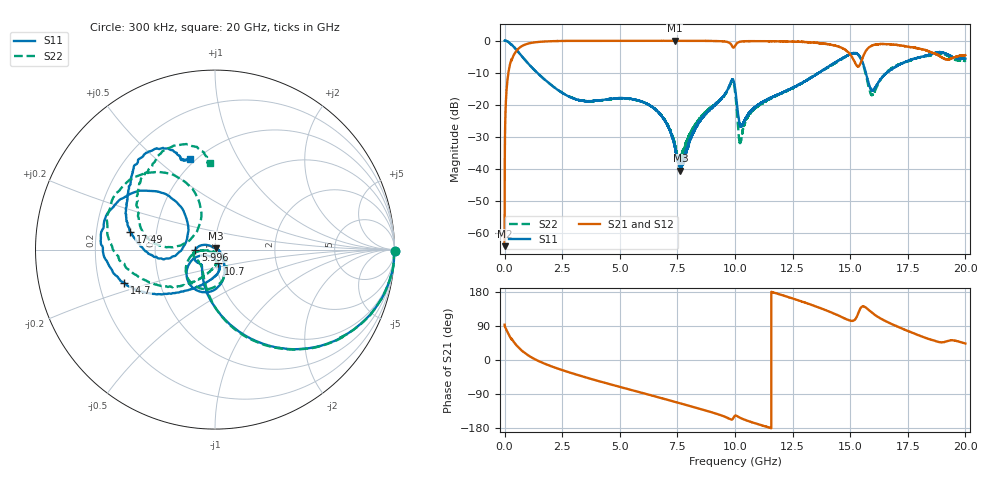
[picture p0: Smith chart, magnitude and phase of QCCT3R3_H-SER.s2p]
!{QCCT3R3}
!Johanson Technology Inc.
!www.johansontechnology.com
!Test Board Conditions:
!Substrate Type  RO4350B
!Substrate Thickness  20 mil
!Substrate Dk  3.66
!TL Type: GCPW
!TL Trace Width  34 mil
!TL Gap  10 mil
!Electrode orientation  Horizontal
!DUT TOPOLOGY	SERIES
!Mounting Pad LxW  26x52 mil
# MHz S  dB  R 50
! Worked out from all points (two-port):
!   20001 points, 300 kHz to 20 GHz, reference 50 ohm
!   highest |S21| = -0.05 dB at 7.375 GHz (marker M1); lowest = -64.3 dB at 300 kHz (marker M2)
!   |S21| within 3 dB of the highest: 530.1 MHz to 14.82 GHz (14.29 GHz wide, 186 % of centre); 15.7 GHz to 18.29 GHz (2.596 GHz wide, 15.3 % of centre)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
!   lowest |S11| = -40.7 dB at 7.63 GHz (marker M3), VSWR 1.02, Z = 50.4 + j0.821 ohm
!   |S11| at or under -10 dB: 1.404 GHz to 13.65 GHz (12.25 GHz wide, 163 % of centre); 15.68 GHz to 16.6 GHz (919.4 MHz wide, 5.7 % of centre)
!   |S22| runs from -37.5 to 0.0 dB; largest |S21 - S12| = 0.018
!   S11 on the Smith chart (normalised r, x): 300 kHz: open; 5.996 GHz: 0.80, -0.00; 10.7 GHz: 1.02, -0.16; 14.7 GHz: 0.31, -0.16; 17.49 GHz: 0.35, +0.09; 20 GHz: 0.47, +0.65
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0.3  0.01 -0.3  -64.26 93.0  -64.31 87.4  0.00 -0.3
125.298  -0.27 -15.9  -12.27 73.8  -12.24 73.8  -0.27 -16.0
431.294  -2.19 -44.4  -4.09 45.2  -4.07 45.2  -2.20 -44.7
1350.28  -9.62 -89.0  -0.53 1.0  -0.53 1.0  -9.62 -89.0
3334.25  -18.76 -129.4  -0.09 -42.4  -0.09 -42.5  -18.74 -134.1
5996.21  -19.20 -179.8  -0.11 -87.2  -0.10 -87.2  -19.16 -174.1
6667.2  -22.37 161.0  -0.09 -98.3  -0.09 -98.2  -22.25 -175.7
7375.189  -32.70 137.2  -0.05 -110.2  -0.06 -110.2  -31.97 -170.4
7630.186  -40.68 61.7  -0.06 -114.5  -0.06 -114.6  -36.40 -83.7
8494.173  -25.06 -43.2  -0.09 -129.3  -0.09 -129.3  -24.14 -42.0
9851.152  -12.46 -98.1  -1.43 -157.2  -1.43 -157.2  -12.95 -101.4
10000.15  -14.76 -147.1  -1.71 -147.1  -1.69 -147.2  -15.96 -159.0
10229.15  -26.72 -125.8  -0.35 -152.7  -0.34 -152.7  -31.73 -117.4
10696.14  -22.03 -76.9  -0.16 -163.6  -0.17 -163.5  -22.52 -83.8
13334.1  -11.43 -123.0  -0.57 145.3  -0.56 145.1  -11.45 -132.0
14703.08  -5.40 -159.9  -2.51 111.2  -2.48 111.3  -5.40 -173.7
15486.07  -5.94 139.3  -6.40 139.4  -6.50 139.1  -6.09 121.2
15950.06  -15.54 159.5  -1.55 124.5  -1.53 124.5  -17.02 143.4
16667.05  -9.63 -172.9  -1.14 98.6  -1.29 98.6  -9.38 174.0
17493.04  -6.33 168.3  -1.92 76.8  -1.94 76.6  -6.57 155.4
18971.01  -3.70 122.6  -5.28 46.5  -5.21 46.6  -4.09 111.4
20000  -5.65 105.7  -4.59 43.5  -4.70 43.6  -6.37 93.3
